FUNCTION FC 101 : VOID
TITLE =One-Shoot Toggle
//Toggle Flip Flop function block
//Usage:
//please assign a bit for each variable, input output plus a bit for a merker need
//for front-reveal detection.
//For infos please contact directly at gabriele_corrieri@hotmail.com.
//
//Copyright and disclaimer:
//This block is get as-is without any warranty.
//This block is public domain and freeware only if this text isn't deleted.
//Copyright PLCForum 2003
//Source build on 16:01 30/12/2002

AUTHOR : Corrieri
FAMILY : Digital
NAME : ToggleFF
VERSION : 0.1


VAR_INPUT
  input : BOOL ;	//T-input
END_VAR
VAR_OUTPUT
  output : BOOL ;	//T-output
  Front_reveal : BOOL ;	//Front reveal merker
END_VAR
VAR_TEMP
  T_clock : BOOL ;	//T-Clock driver
END_VAR
BEGIN
NETWORK
TITLE =Toggle Flip Flop
//Toggle Flip Flop is contained all in this segment.
      U     #input;
      FP    #Front_reveal;
      =     #T_clock;

      U     #T_clock;
      UN    #output;
      SPBN  ns;
      S     #output;
      SPA   nr;

ns:   NOP   0;
      U     #T_clock;
      U     #output;
      SPBN  nr;
      R     #output;

nr:   NOP   0;
      BEA   ;
END_FUNCTION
